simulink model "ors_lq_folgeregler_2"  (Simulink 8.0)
settings: Solver=ode45  SolverMode=SingleTasking  StartTime=0.0  StopTime=10  FixedStep=0.01  MaxStep=0.01  RelTol=1e-3  AbsTol=1e-3
undefined symbols (not defined in the file or in its folder): k, k_s

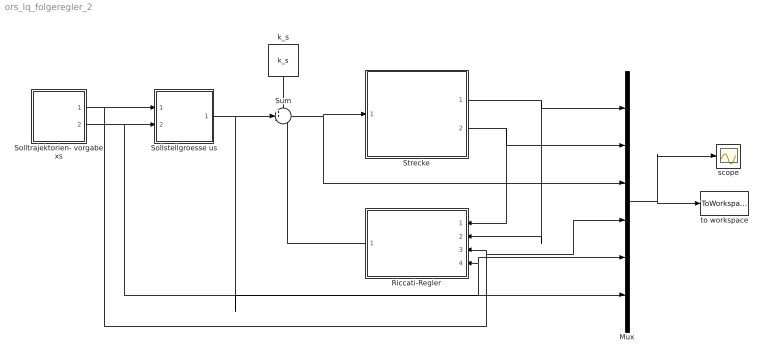
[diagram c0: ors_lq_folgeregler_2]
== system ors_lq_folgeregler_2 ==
  Mux : Mux  Inputs=6
  Riccati-Regler : Subsystem
  Sollstellgroesse us : Subsystem
  Solltrajektorien- vorgabe xs : Subsystem
  Strecke : Subsystem
  Sum : Sum  Inputs=++-
  k_s : Constant  Value=k_s
  scope : Scope
  to workspace : ToWorkspace  VariableName=simout  SampleTime=-1  SaveFormat=Structure With Time
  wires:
  Strecke/1(x1) -> Riccati-Regler/2(x1), Mux/1
  Strecke/2(x2) -> Riccati-Regler/1(x2), Mux/2
  Mux/1 -> to workspace/1, scope/1
  Solltrajektorien- vorgabe xs/1(x1s) -> Sollstellgroesse us/1(x1s), Riccati-Regler/3(x1s), Mux/4
  Solltrajektorien- vorgabe xs/2(x2s) -> Sollstellgroesse us/2(x2s), Riccati-Regler/4(x2s), Mux/5
  Sollstellgroesse us/1(us) -> Mux/6, Sum/2
  Sum/1 -> Strecke/1(u), Mux/3
  Riccati-Regler/1(-du-R^(-1)*B'*p) -> Sum/3
  k_s/1 -> Sum/1

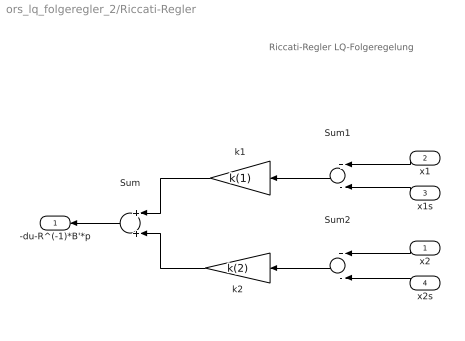
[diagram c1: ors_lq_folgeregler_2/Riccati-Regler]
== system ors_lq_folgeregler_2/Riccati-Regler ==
  note: Riccati-Regler LQ-Folgeregelung
  x2 : Inport
  x1 : Inport  Port=2
  x1s : Inport  Port=3
  x2s : Inport  Port=4
  Sum : Sum
  Sum1 : Sum  Inputs=+-
  Sum2 : Sum  Inputs=+-
  k1 : Gain  Gain=k(1)
  k2 : Gain  Gain=k(2)
  -du-R^(-1)*B'*p : Outport  InitialOutput=0
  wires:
  Sum1/1 -> k1/1
  Sum2/1 -> k2/1
  x2/1 -> Sum2/1
  Sum/1 -> -du-R^(-1)*B'*p/1
  k2/1 -> Sum/2
  k1/1 -> Sum/1
  x1/1 -> Sum1/1
  x1s/1 -> Sum1/2
  x2s/1 -> Sum2/2

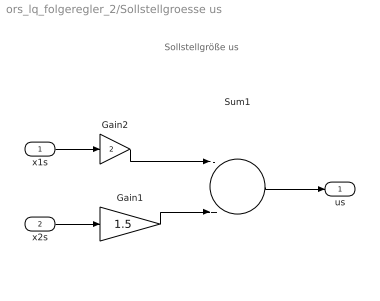
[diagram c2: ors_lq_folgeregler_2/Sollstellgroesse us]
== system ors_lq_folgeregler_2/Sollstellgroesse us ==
  note: Sollstellgröße us
  x1s : Inport
  x2s : Inport  Port=2
  Gain1 : Gain  Gain=1.5
  Gain2 : Gain  Gain=2
  Sum1 : Sum  Inputs=-+
  us : Outport  InitialOutput=0
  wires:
  Gain2/1 -> Sum1/1
  Gain1/1 -> Sum1/2
  Sum1/1 -> us/1
  x1s/1 -> Gain2/1
  x2s/1 -> Gain1/1

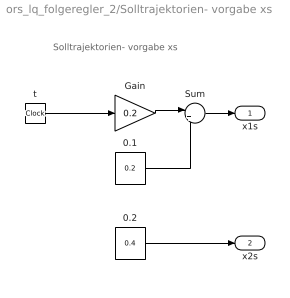
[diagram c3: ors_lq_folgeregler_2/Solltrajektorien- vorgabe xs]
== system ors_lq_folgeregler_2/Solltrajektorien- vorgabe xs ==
  note: Solltrajektorien- vorgabe xs
  0.1 : Constant  Value=0.2
  0.2 : Constant  Value=0.4
  Gain : Gain  Gain=0.2
  Sum : Sum  Inputs=|++
  t : Clock
  x1s : Outport  InitialOutput=0
  x2s : Outport  Port=2  InitialOutput=0
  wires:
  0.2/1 -> x2s/1
  t/1 -> Gain/1
  Gain/1 -> Sum/1
  Sum/1 -> x1s/1
  0.1/1 -> Sum/2

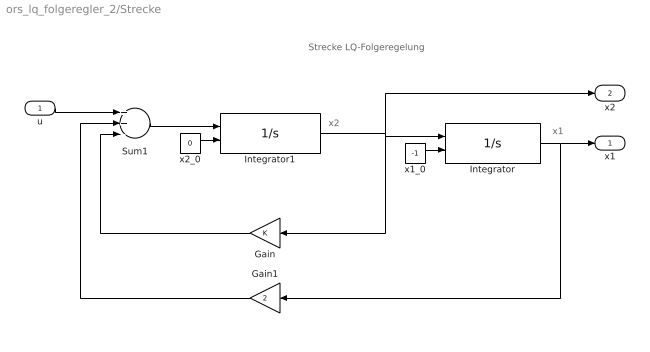
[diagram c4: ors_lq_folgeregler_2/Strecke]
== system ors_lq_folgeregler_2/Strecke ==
  note: x1
  note: x2
  note: Strecke LQ-Folgeregelung
  u : Inport
  Gain : Gain
  Gain1 : Gain  Gain=2
  Integrator : Integrator  InitialConditionSource=external
  Integrator1 : Integrator  InitialConditionSource=external
  Sum1 : Sum  Inputs=++-
  x1_0 : Constant  Value=-1
  x2_0 : Constant  Value=0
  x1 : Outport  InitialOutput=0
  x2 : Outport  Port=2  InitialOutput=0
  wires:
  Integrator1/1 -> Integrator/1, Gain/1, x2/1
  Sum1/1 -> Integrator1/1
  Gain/1 -> Sum1/3
  Gain1/1 -> Sum1/2
  u/1 -> Sum1/1
  Integrator/1 -> Gain1/1, x1/1
  x2_0/1 -> Integrator1/2
  x1_0/1 -> Integrator/2
